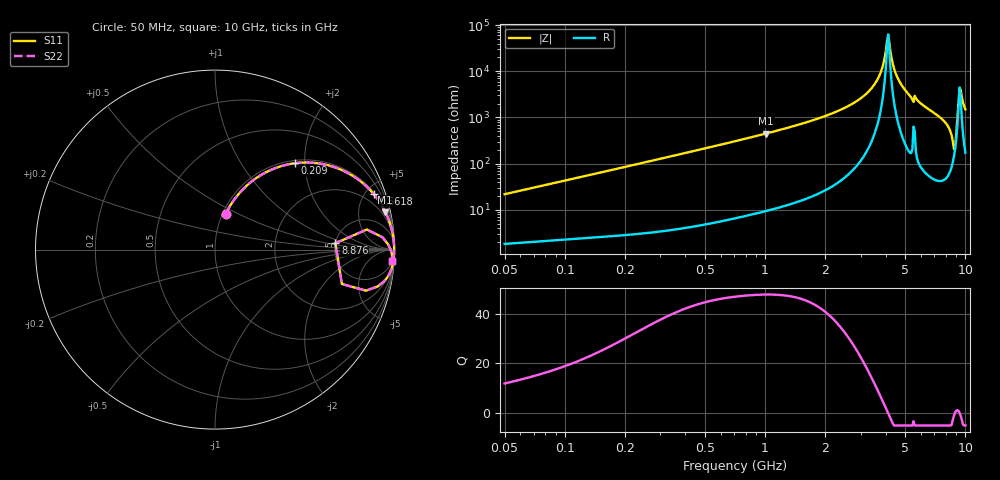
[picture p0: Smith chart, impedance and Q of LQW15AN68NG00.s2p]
!Murata Part Number: LQW15AN68NG00
!These Parameters are Measured in Series Mode Connection
!  o--[Z]--o
!Port1  Port2
!  o-------o
!Freq. Start=50[MHz] Stop=10[GHz], 401[Steps]
# Hz S RI R 50
!Freq.(Hz)	S 11(Real)	S 11(Imag)	S 21(Real)	S 21(Imag)	S 12(Real)	S 12(Imag)	S 22(Real)	S 22(Imag)
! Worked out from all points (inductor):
!   401 points, 50 MHz to 10 GHz, reference 50 ohm
!   read as one part in series: L = 68.6 nH near 51.34 MHz
!   highest Q = 47.7 at 1.011 GHz (marker M1), where L = 70.7 nH
!   self-resonance near 4.063 GHz
!   S11 on the Smith chart (normalised r, x): 50 MHz: 1.04, +0.43; 209 MHz: 1.06, +1.78; 661.8 MHz: 1.12, +5.70; 8.876 GHz: 5.01, +0.64; 10 GHz: 4, -30
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5e7  0.0604 0.1999  0.9396 -0.1999  0.9396 -0.1999  0.0604 0.1999
1.214486e8  0.2228 0.3936  0.7772 -0.3936  0.7772 -0.3936  0.2228 0.3936
2.09049e8  0.4433 0.4808  0.5567 -0.4808  0.5567 -0.4808  0.4433 0.4808
2.949953e8  0.6085 0.4749  0.3915 -0.4749  0.3915 -0.4749  0.6085 0.4749
6.617929e8  0.8854 0.308  0.1146 -0.308  0.1146 -0.308  0.8854 0.308
7.071068e8  0.8983 0.2918  0.1017 -0.2918  0.1017 -0.2918  0.8983 0.2918
1.011124e9  0.9488 0.2101  0.0512 -0.2101  0.0512 -0.2101  0.9488 0.2101
1.717543e9  0.9842 0.114  0.0158 -0.114  0.0158 -0.114  0.9842 0.114
2.521925e9  0.9945 0.06  0.00551 -0.06  0.00551 -0.06  0.9945 0.06
3.243629e9  0.9975 0.0287  0.00248 -0.0287  0.00248 -0.0287  0.9975 0.0287
3.703027e9  0.9982 0.0128  0.00175 -0.0128  0.00175 -0.0128  0.9982 0.0128
3.853138e9  0.9984 0.00794  0.00165 -0.00794  0.00165 -0.00794  0.9984 0.00794
4.062795e9  0.9984 0.00149  0.00158 -0.00149  0.00158 -0.00149  0.9984 0.00149
4.171863e9  0.9984 -0.00177  0.00158 0.00177  0.00158 0.00177  0.9984 -0.00177
4.457516e9  0.9983 -0.01  0.0017 0.01  0.0017 0.01  0.9983 -0.01
4.955797e9  0.9977 -0.024  0.00227 0.024  0.00227 0.024  0.9977 -0.024
7.775012e9  0.981 -0.1134  0.019 0.1134  0.019 0.1134  0.981 -0.1134
8.530394e9  0.9066 -0.2051  0.0934 0.2051  0.0934 0.2051  0.9066 -0.2051
8.876195e9  0.6709 0.0353  0.3291 -0.0353  0.3291 -0.0353  0.6709 0.0353
9.359165e9  0.978 0.000665  0.022 -0.000665  0.022 -0.000665  0.978 0.000665
9.610418e9  0.9867 -0.0345  0.0133 0.0345  0.0133 0.0345  0.9867 -0.0345
1e10  0.9882 -0.0647  0.0118 0.0647  0.0118 0.0647  0.9882 -0.0647
